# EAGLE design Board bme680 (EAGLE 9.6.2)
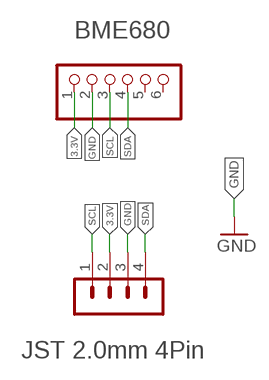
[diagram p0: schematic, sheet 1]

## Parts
JP1  PINHD-1X6  [1X06]
JST2.0MM4PIN  B4B-PH-K-S  [B4B-PH-K-S]

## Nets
3.3V: JP1.1 JST2.0MM4PIN.2
GND: JP1.2 JST2.0MM4PIN.3
SCL: JP1.3 JST2.0MM4PIN.1
SDA: JP1.4 JST2.0MM4PIN.4
Unconnected: JP1.5 JP1.6

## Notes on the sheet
- BME680
- JST 2.0mm 4Pin

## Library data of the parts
JP1 = pinhead:PINHD-1X6: PIN HEADER
JST2.0MM4PIN = con-JSTPH:B4B-PH: JST PH series header 2.00mm pitch disconnectable crimp style connectors, vertical (side entry type), 4 pins

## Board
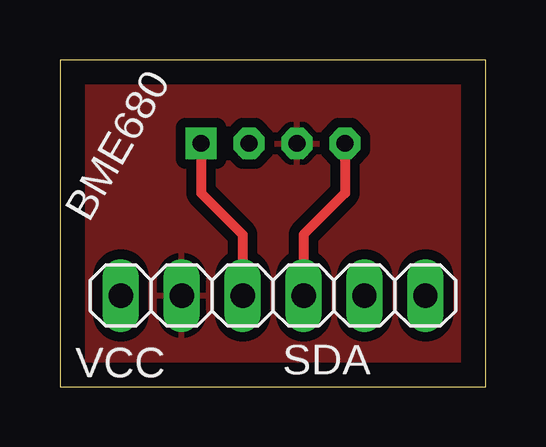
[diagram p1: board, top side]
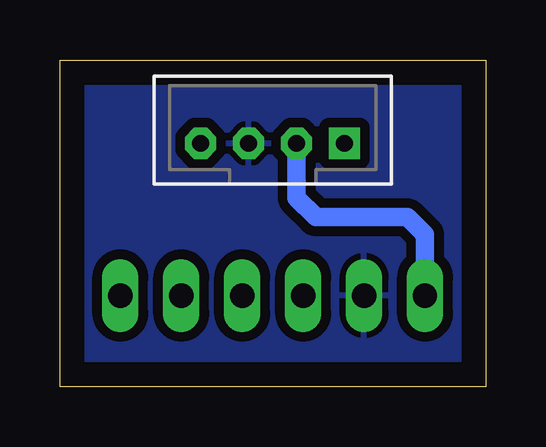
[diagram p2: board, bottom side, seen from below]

Size 17.76 x 13.64 mm. Coordinates in mm from the lower left corner, seen from the top.
Outline: 0,0 17.76,0 17.76,13.64 0,13.64 0,0
Copper layers (1*16): Top 0.035mm / dielectric 1.5mm / Bottom 0.035mm
Design rules "default": minimum track width 6mil, minimum drill 0.35mm, track to track 6mil, track to pad 6mil, pad to pad 6mil, via to via 6mil, smd to smd 6mil, copper to edge 40mil, drill to drill 6mil, minimum pad ring 10mil, minimum via ring 8mil, stop-mask expansion 4mil, vias tented up to drill 0mil, thermal gap 10mil

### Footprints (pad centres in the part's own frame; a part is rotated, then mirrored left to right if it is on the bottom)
1X06 = drill 1.016 long: 1 -6.35,0; 2 -3.81,0; 3 -1.27,0; 4 1.27,0; 5 3.81,0; 6 6.35,0
B4B-PH-K-S = drill 0.7 pad 1.3 square: 1 3,0 | drill 0.7 pad 1.3 octagon: 2 1,0; 3 -1,0; 4 -3,0

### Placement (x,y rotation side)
JP1  8.89,3.81 0 top
JST2.0MM4PIN  8.89,10.16 0 bottom

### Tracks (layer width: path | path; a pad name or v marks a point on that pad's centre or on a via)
3.3V
  Bottom 0.762: JST2.0MM4PIN.2 7.89,7.89 7.09,7.09 3.28,7.09 2.54,6.35 JP1.1
GND
  pour Bottom (isolate 0.406): 0,13.97 17.78,13.97 17.78,0 0,0
  pour Top (isolate 0.406): 0,13.97 17.78,13.97 17.78,0 0,0
SCL
  Top 0.406: JST2.0MM4PIN.1 5.89,8.08 7.62,6.35 JP1.3
SDA
  Top 0.406: JST2.0MM4PIN.4 11.89,8.08 10.16,6.35 JP1.4

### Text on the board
tPlace: BME680 | VCC | SDA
